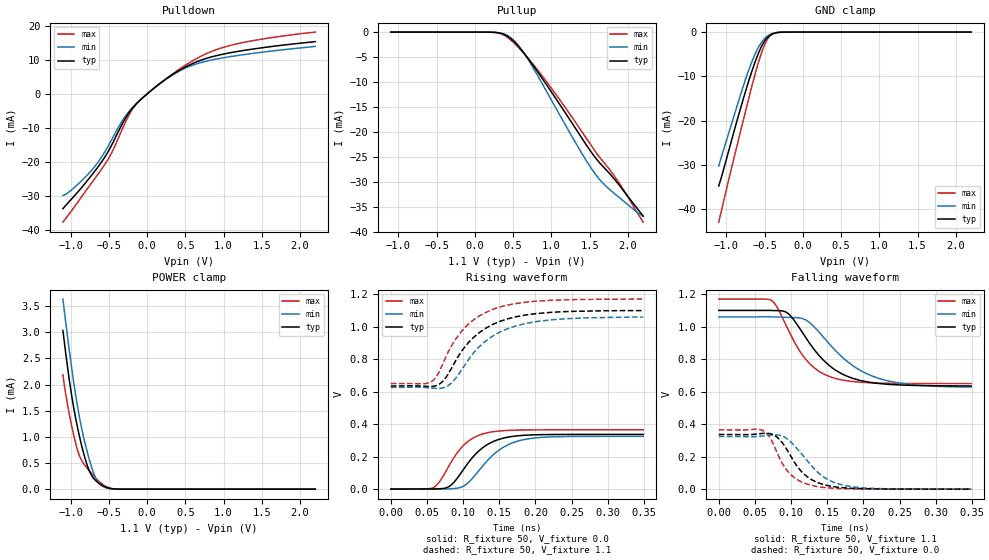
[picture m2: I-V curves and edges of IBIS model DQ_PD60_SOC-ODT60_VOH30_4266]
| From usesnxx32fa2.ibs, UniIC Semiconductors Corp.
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| DQ_PD60_SOC-ODT60_VOH30_4266
| (60 Ohm Pulldown, 60 Ohm System ODT Setting, VOH=VDDQ/3.0, 3200-4266Mbps)
[Model]   DQ_PD60_SOC-ODT60_VOH30_4266
Model_type   I/O
Vinl = 123.333mV
Vinh = 243.333mV
Vmeas = 183.333mV
Vref = 0.0mV
Cref = 0.0pF
Rref = 60.000Ohm
|   typ   min   max
|C_comp   0.834pF   0.784pF   0.884pF
C_comp_pullup   0.4170pF   0.3920pF   0.4420pF
C_comp_pulldown   0.4170pF   0.3920pF   0.4420pF
| Note: C_comp changes when the ODT circuit is enabled.
[Model Spec]
| Input threshold voltage corners
Vinl   0.1233V   0.1167V   0.1350V
Vinh   0.2433V   0.2367V   0.2550V
| Measurement voltage corners
Vmeas   0.1833V   0.1767V   0.1950V
| Timing spec test load voltage corners
Vref   0.0000V   0.0000V   0.0000V
| Dynamic Overshoot Parameters from LPDDR4 Specification
D_overshoot_ampl_h   0.30   NA   NA
D_overshoot_ampl_l   0.30   NA   NA
D_overshoot_area_h   0.1n   NA   NA
D_overshoot_area_l   0.1n   NA   NA
[Voltage Range]   1.1000V   1.0600V   1.1700V
[Pullup Reference]   1.1000V   1.0600V   1.1700V
| Junction Temperature (Ambient temp is 35C typ 95C min -40C max)
[Temperature Range]   50.0   110.0   -40.0
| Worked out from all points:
|   slope of the pulldown table from 0 to 0.165 V, typ, clamps not added: 54.9 ohm
|   slope of the pullup table from 0 to 0.165 V, typ, clamps not added: 19.5 kohm
|   GND clamp passes 1 mA (typ) near -0.45 V on its own axis
|   POWER clamp passes 1 mA (typ) near -0.88 V on its own axis
|   rising waveform, R_fixture 50, V_fixture 0.0: 20-80 % time 39.8ps typ, 43.7ps min, 34.9ps max; typ from 0 V to 0.337 V
|   falling waveform, R_fixture 50, V_fixture 1.1: 20-80 % time 53.7ps typ, 65.5ps min, 43.2ps max; typ from 1.1 V to 0.635 V
|   rising waveform, R_fixture 50, V_fixture 1.1: 20-80 % time 55.8ps typ, 59ps min, 52.2ps max; typ from 0.635 V to 1.1 V
|   falling waveform, R_fixture 50, V_fixture 0.0: 20-80 % time 34.7ps typ, 42.3ps min, 30ps max; typ from 0.337 V to 0.001 V
[Pulldown]
|   Voltage   I(typ)   I(min)   I(max)
-1.1V     -33.69mA   -29.81mA   -37.65mA
-918.5mV  -29.13mA   -26.82mA   -32.19mA
-684.2mV  -22.7mA    -21.33mA   -24.89mA
-473mV    -15.47mA   -13.89mA   -17.74mA
-321.2mV  -8.698mA   -7.822mA   -10.19mA
-179.3mV  -3.868mA   -3.748mA   -4.114mA
-60.5mV   -1.212mA   -1.204mA   -1.195mA
262.9mV   4.608mA    4.54mA     4.696mA
589.6mV   8.859mA    8.394mA    9.639mA
969.1mV   11.55mA    10.5mA     13.47mA
1.448V    13.37mA    12.09mA    15.89mA
2.2V      15.34mA    13.95mA    18.15mA
[GND Clamp]
|   Voltage   I(typ)   I(min)   I(max)
-1.1V     -34.74mA   -30.22mA   -42.91mA
-944.9mV  -25.23mA   -21.44mA   -31.55mA
-796.4mV  -16.11mA   -13.14mA   -21.19mA
-723.8mV  -11.93mA   -9.349mA   -16.1mA
-664.4mV  -8.736mA   -6.578mA   -12.07mA
-591.8mV  -5.255mA   -3.789mA   -7.493mA
-519.2mV  -2.565mA   -1.832mA   -3.66mA
-466.4mV  -1.294mA   -942uA     -1.691mA
-413.6mV  -564.7uA   -417.1uA   -621.5uA
-354.2mV  -178.2uA   -134.5uA   -160uA
-251.9mV  -13.34uA   -11.9uA    -7.88uA
2.2V      0A         0A         0A
[Pullup]
|   Voltage   I(typ)   I(min)   I(max)
-1.1V     4.184uA    6.447uA    1.886uA
233.2mV   -32.57uA   -32.57uA   -33.77uA
335.5mV   -227.6uA   -188.6uA   -312.9uA
434.5mV   -925.6uA   -756.8uA   -1.171mA
556.6mV   -2.656mA   -2.458mA   -2.871mA
695.2mV   -5.309mA   -5.489mA   -5.24mA
1.078V    -13.79mA   -15.78mA   -12.9mA
1.411V    -21.57mA   -24.66mA   -20.25mA
1.566V    -25.01mA   -28.3mA    -23.76mA
1.698V    -27.32mA   -30.67mA   -26.36mA
1.873V    -30.42mA   -32.98mA   -29.96mA
2.2V      -36.89mA   -36.88mA   -38.1mA
[POWER Clamp]
|   Voltage   I(typ)   I(min)   I(max)
-1.1V     3.033mA    3.633mA    2.184mA
-1.044V   2.381mA    2.967mA    1.653mA
-981.2mV  1.752mA    2.275mA    1.183mA
-908.6mV  1.178mA    1.582mA    748.9uA
-849.2mV  799uA      1.125mA    535.5uA
-773.3mV  420.8uA    665.2uA    384.1uA
-710.6mV  232.2uA    359.1uA    273.1uA
-657.8mV  146.8uA    178.9uA    190.7uA
-595.1mV  80.77uA    68.29uA    109.3uA
-496.1mV  20.06uA    12.31uA    25.72uA
-390.5mV  2.036uA    1.382uA    1.767uA
2.2V      0A         0A         0A
[Ramp]
|   typ   min   max
| 20% - 80%
dV/dt_r   201.83m/39.76p   194.56m/43.73p   218.89m/34.90p
dV/dt_f   278.76m/53.65p   259.05m/65.50p   312.07m/43.27p
| 25% - 75%
|dV/dt_r   168.19m/31.74p   162.14m/34.85p   182.41m/27.73p
|dV/dt_f   232.30m/42.76p   215.87m/52.22p   260.06m/34.39p
R_load = 50
[Rising Waveform]
R_fixture = 50
V_fixture = 0.0
|   Time   V(typ)   V(min)   V(max)
0s        464.8uV    400.6uV    339.4uV
58ps      324.4uV    15.1uV     7.762mV
67ps      1.966mV    -349.5uV   44.26mV
79ps      12.18mV    1.022mV    132mV
89ps      50.67mV    3.933mV    205.8mV
103ps     137.4mV    25.18mV    279.4mV
132ps     270.2mV    168.1mV    345.6mV
156ps     314.3mV    258.7mV    360mV
189ps     332.6mV    309.1mV    364.4mV
349ps     336.8mV    324.7mV    365.2mV
[Falling Waveform]
R_fixture   = 50
V_fixture   = 1.1
V_fixture_min = 1.06
V_fixture_max = 1.17
|   Time   V(typ)   V(min)   V(max)
0s        1.1V       1.06V      1.17V
74ps      1.1V       1.06V      1.158V
96ps      1.081V     1.057V     981.3mV
119ps     941.5mV    1.044V     806.6mV
136ps     837.1mV    980.3mV    733.5mV
158ps     743.3mV    869.1mV    686mV
189ps     677mV      749.4mV    660.9mV
226ps     648.4mV    675.8mV    652.6mV
274ps     638.2mV    640.6mV    650.3mV
349ps     635.4mV    628.2mV    649.9mV
[Rising Waveform]
R_fixture   = 50
V_fixture   = 1.1
V_fixture_min = 1.06
V_fixture_max = 1.17
|   Time   V(typ)   V(min)   V(max)
0s        635mV      626.1mV    649.8mV
55ps      631.5mV    622.4mV    659.3mV
64ps      639.2mV    619.6mV    700.1mV
77ps      692.5mV    631.4mV    822.9mV
90ps      793.2mV    684.1mV    925.3mV
106ps     895mV      789.5mV    1.01V
125ps     972.1mV    888.2mV    1.073V
147ps     1.026V     957.7mV    1.116V
213ps     1.085V     1.038V     1.16V
349ps     1.099V     1.059V     1.17V
[Falling Waveform]
R_fixture = 50
V_fixture = 0.0
|   Time   V(typ)   V(min)   V(max)
0s        336.9mV    324.8mV    365.2mV
58ps      342.3mV    326.4mV    366.5mV
67ps      344.2mV    331.2mV    339.7mV
76ps      334.2mV    334.9mV    273.5mV
97ps      223.7mV    301.7mV    102.1mV
112ps     121.1mV    230.9mV    50.24mV
128ps     60.02mV    145.6mV    23.85mV
151ps     22.16mV    59.28mV    8.458mV
183ps     6.007mV    16.13mV    2.206mV
349ps     542.3uV    526.3uV    362.3uV
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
